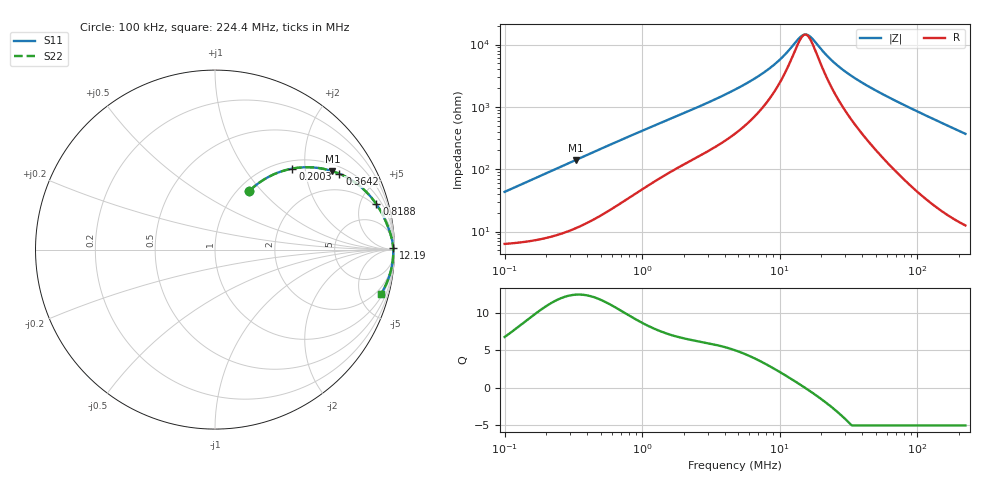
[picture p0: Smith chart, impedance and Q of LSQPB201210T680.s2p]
! LSQPB201210T680  S-PARAMETER MODEL  ( General Type )
! Model Generated by TAIYO YUDEN Corporation (http://www.ty-top.com)
! Version 2.0
! TAIYO YUDEN Control No. 100810NF18SB-HKC
! Copyright(c) 2007 TAIYO YUDEN CO.,LTD. All Rights Reserved.
! Product Description (link to TY-COMPAS)
! https://ds.yuden.co.jp/TYCOMPAS/or/detail?pn=LSQPB201210T680M&u=M
! Products Name : Inductors
! Characteristics :
!  Inductance : 68 uH , SRF(min) : 6.5 MHz , DC Resistance(max) : 7.54 Ohm
!  Rated Current : Saturation :100 mA , Temp Rise : 110 mA (40 degC)
!  Case Size : 2.0 x 1.25 / 0.079 x 0.049 [mm/inch] , Thickness : 1.0 / 0.04 [mm/inch]
!  (Conditions: Temperature = 25 degC , DC Bias Current/Voltage = 0A / 0V)
! External Node Assignments :
!  1  o---GGG---o  2
! GND o---------o GND
! Frequency Range : 0.1MHz  -  224.402193MHz  [ 402 STEP ]
# MHz S RI R 50
! Freq[MHz].  S11 Real  S11 Imag  S21 Real  S21 Imag  S12 Real  S12 Imag  S22 Real  S22 Imag
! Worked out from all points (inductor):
!   401 points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, 100 kHz to 224.4 MHz, reference 50 ohm
!   read as one part in series: L = 68.1 uH near 103.9 kHz
!   highest Q = 12.4 at 330.7 kHz (marker M1), where L = 67.8 uH
!   self-resonance near 15.07 MHz
!   S11 on the Smith chart (normalised r, x): 100 kHz: 1.13, +0.86; 200.3 kHz: 1.16, +1.71; 364.2 kHz: 1.25, +3.10; 818.8 kHz: 1.71, +6.80; 12.19 MHz: open; 224.4 MHz: 1.25, -7.39
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0.1  0.1906 0.3258  0.8094 -0.3258  0.8094 -0.3258  0.1906 0.3258
0.138809  0.2847 0.3976  0.7153 -0.3976  0.7153 -0.3976  0.2847 0.3976
0.200259  0.4309 0.4513  0.5691 -0.4513  0.5691 -0.4513  0.4309 0.4513
0.330681  0.6543 0.437  0.3457 -0.437  0.3457 -0.437  0.6543 0.437
0.364164  0.6929 0.4227  0.3071 -0.4227  0.3071 -0.4227  0.6929 0.4227
0.53561  0.8171 0.3455  0.1829 -0.3455  0.1829 -0.3455  0.8171 0.3455
0.818757  0.8989 0.2536  0.1011 -0.2536  0.1011 -0.2536  0.8989 0.2536
1.326154  0.9459 0.1699  0.0541 -0.1699  0.0541 -0.1699  0.9459 0.1699
2.813968  0.9777 0.0867  0.0223 -0.0867  0.0223 -0.0867  0.9777 0.0867
4.737111  0.9872 0.0506  0.0128 -0.0506  0.0128 -0.0506  0.9872 0.0506
8.288253  0.9916 0.0232  0.00839 -0.0232  0.00839 -0.0232  0.9916 0.0232
10.24746  0.9924 0.0147  0.0076 -0.0147  0.0076 -0.0147  0.9924 0.0147
12.1903  0.9928 0.00827  0.00717 -0.00827  0.00717 -0.00827  0.9928 0.00827
14.78393  0.9931 0.00133  0.00687 -0.00133  0.00687 -0.00133  0.9931 0.00133
15.96983  0.9932 -0.00143  0.0068 0.00143  0.0068 0.00143  0.9932 -0.00143
17.25085  0.9933 -0.0042  0.00674 0.0042  0.00674 0.0042  0.9933 -0.0042
22.59938  0.9933 -0.0142  0.00672 0.0142  0.00672 0.0142  0.9933 -0.0142
28.48573  0.9931 -0.0237  0.00692 0.0237  0.00692 0.0237  0.9931 -0.0237
39.54085  0.9923 -0.0395  0.00771 0.0395  0.00771 0.0395  0.9923 -0.0395
62.8214  0.9892 -0.0696  0.0108 0.0696  0.0108 0.0696  0.9892 -0.0696
121.0445  0.9738 -0.139  0.0262 0.139  0.0262 0.139  0.9738 -0.139
224.4022  0.9246 -0.2476  0.0754 0.2476  0.0754 0.2476  0.9246 -0.2476
